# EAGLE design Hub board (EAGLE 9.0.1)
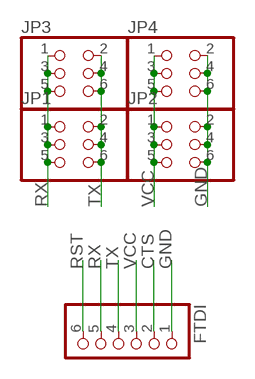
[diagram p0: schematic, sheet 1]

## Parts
FTDI  PINHD-1X6  [1X06]
JP1  PINHD-2X3-SMD  [2X03SMD]
JP2  PINHD-2X3-SMD  [2X03SMD]
JP3  PINHD-2X3-SMD  [2X03SMD]
JP4  PINHD-2X3-SMD  [2X03SMD]

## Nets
CTS: FTDI.2
GND: FTDI.1 JP2.2 JP2.4 JP2.6 JP4.2 JP4.4 JP4.6
RST: FTDI.6
RX: FTDI.5 JP1.1 JP1.3 JP1.5 JP3.1 JP3.3 JP3.5
TX: FTDI.4 JP1.2 JP1.4 JP1.6 JP3.2 JP3.4 JP3.6
VCC: FTDI.3 JP2.1 JP2.3 JP2.5 JP4.1 JP4.3 JP4.5

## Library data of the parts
FTDI = adafruit:PINHD-1X6: PIN HEADER
JP1-JP4 = fab:PINHD-2X3-SMD: PIN HEADER

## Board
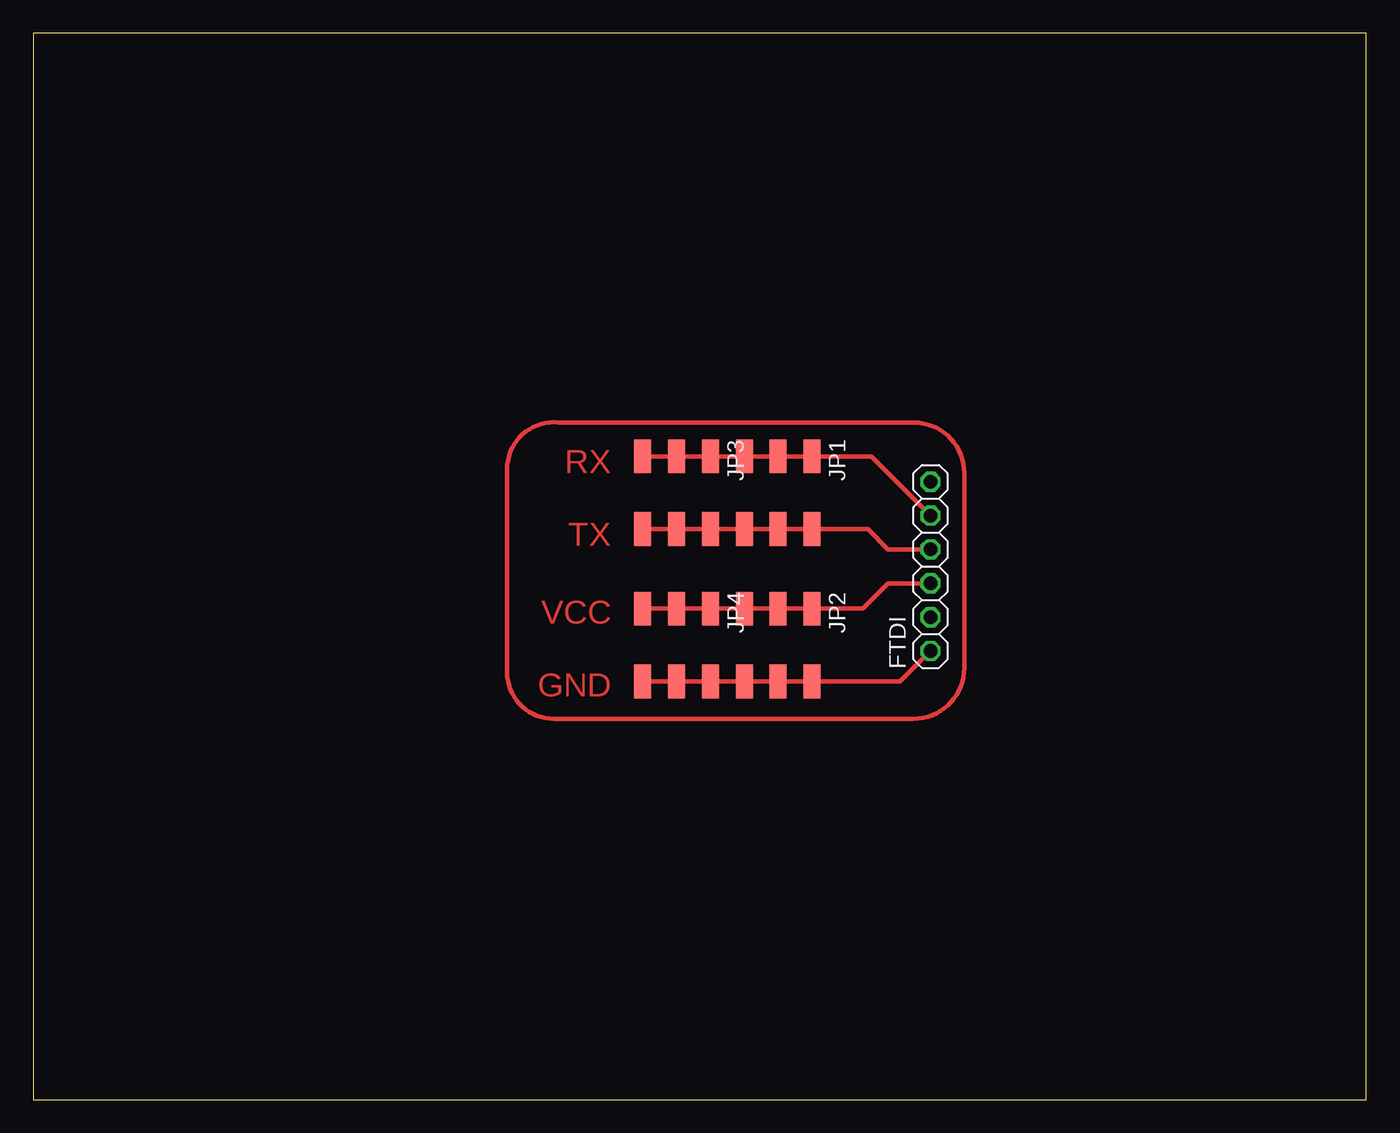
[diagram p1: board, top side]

Size 100 x 80 mm. Coordinates in mm from the lower left corner, seen from the top.
Outline: 0,0 100,0 100,80 0,80 0,0
Copper layers (1*16): Top 0.035mm / dielectric 1.5mm / Bottom 0.035mm
Design rules "default *": minimum track width 14mil, minimum drill 0.35mm, track to track 14mil, track to pad 14mil, pad to pad 14mil, via to via 14mil, smd to smd 14mil, copper to edge 40mil, drill to drill 6mil, minimum pad ring 10mil, minimum via ring 8mil, stop-mask expansion 4mil, vias tented up to drill 0mil, thermal gap 10mil

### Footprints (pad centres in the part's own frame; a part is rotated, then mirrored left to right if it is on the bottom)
1X06 = drill 1.016 octagon: 1 -6.35,0; 2 -3.81,0; 3 -1.27,0; 4 1.27,0; 5 3.81,0; 6 6.35,0
2X03SMD = smd 2.54 x 1.27: 1 -2.54,2.54; 2 2.92,2.54; 3 -2.54,0; 4 2.92,0; 5 -2.54,-2.54; 6 2.92,-2.54

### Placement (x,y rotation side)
FTDI  67.31,40.01 90 top
JP1  55.88,45.72 270 top
JP2  55.88,34.29 270 top
JP3  48.26,45.72 270 top
JP4  48.26,34.29 270 top

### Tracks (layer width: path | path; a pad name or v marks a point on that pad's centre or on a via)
GND
  Top 0.356: FTDI.1 65.03,31.37 JP2.2 JP2.4 JP2.6 JP4.2 JP4.4 JP4.6
N$1
  Top 0.356: 69.85,32.38 69.85,46.99 arc90 66.04,50.8 39.37,50.8 arc90 35.56,47.62 35.56,31.75 arc90 39.37,28.57 66.04,28.57 arc90 69.85,32.38
RX
  Top 0.356: FTDI.5 62.87,48.26 JP1.1 JP1.3 JP1.5 JP3.1 JP3.3 JP3.5
TX
  Top 0.356: FTDI.4 64.14,41.27 62.61,42.8 JP1.2 JP1.4 JP1.6 JP3.2 JP3.4 JP3.6
VCC
  Top 0.356: JP4.5 JP4.3 JP4.1 JP2.5 JP2.3 JP2.1 62.23,36.83 64.14,38.73 FTDI.3

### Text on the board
Top: RX | TX | VCC | GND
